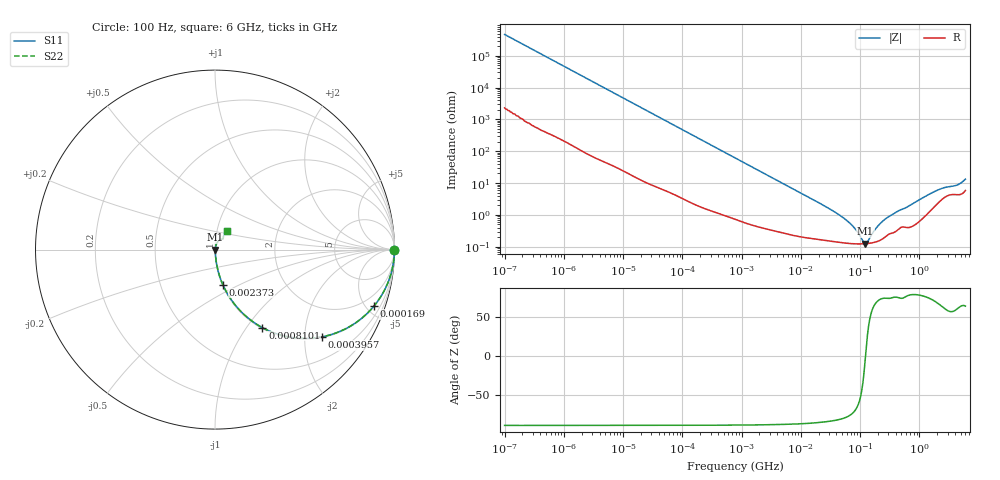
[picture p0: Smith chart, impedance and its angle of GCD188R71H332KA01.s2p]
!Murata Part Number: GCD188R71H332KA01
!These Parameters are Measured in Series Mode Connection
!Data Generated on Jan 08, 2026
!  o--ll--o
!Port1  Port2
!  o------o
!Operation Temp=25[degC], DC Bias Voltage=0[V]
!Freq. Start=100[Hz] Stop=6[GHz] 401[Steps]
# Hz S RI R 50
!Freq.(Hz) S11(Real) S11(Imag) S21(Real) S21(Imag) S12(Real) S12(Imag) S22(Real) S22(Imag)
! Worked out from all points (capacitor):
!   401 points, 100 Hz to 6 GHz, reference 50 ohm
!   read as one part in series: C = 3.4 nF near 109 Hz
!   lowest |Z| = 124 mohm at 122 MHz (marker M1)
!   series resonance near 123.7 MHz, so ESL is about 490 pH
!   S11 on the Smith chart (normalised r, x): 100 Hz: open; 169 kHz: 1.04, -5.66; 395.7 kHz: 1.02, -2.42; 810.1 kHz: 1.01, -1.19; 2.373 MHz: 1.01, -0.41; 6 GHz: 1.12, +0.24
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100  1 -0.000214  1.1e-06 0.000214  1.1e-06 0.000214  1 -0.000214
2008  1 -0.00426  3.67e-05 0.00426  3.67e-05 0.00426  1 -0.00426
40335  0.9924 -0.0842  0.00764 0.0842  0.00764 0.0842  0.9924 -0.0842
169018  0.8871 -0.3129  0.1129 0.3129  0.1129 0.3129  0.8871 -0.3129
395726  0.5941 -0.4864  0.4059 0.4864  0.4059 0.4864  0.5941 -0.4864
774597  0.2811 -0.4437  0.7189 0.4437  0.7189 0.4437  0.2811 -0.4437
810067  0.2637 -0.4347  0.7363 0.4347  0.7363 0.4347  0.2637 -0.4347
1325623  0.1207 -0.3188  0.8793 0.3188  0.8793 0.3188  0.1207 -0.3188
2372521  0.0434 -0.1947  0.9566 0.1947  0.9566 0.1947  0.0434 -0.1947
5311619  0.0109 -0.0906  0.9891 0.0906  0.9891 0.0906  0.0109 -0.0906
1.555665e7  0.00276 -0.0311  0.9972 0.0311  0.9972 0.0311  0.00276 -0.0311
3.64232e7  0.0016 -0.0126  0.9984 0.0126  0.9984 0.0126  0.0016 -0.0126
5.960426e7  0.00133 -0.00654  0.9987 0.00654  0.9987 0.00654  0.00133 -0.00654
8.154455e7  0.00124 -0.00354  0.9988 0.00354  0.9988 0.00354  0.00124 -0.00354
1.115611e8  0.00123 -0.00086  0.9988 0.00086  0.9988 0.00086  0.00123 -0.00086
1.220122e8  0.00124 -0.000115  0.9988 0.000115  0.9988 0.000115  0.00124 -0.000115
1.334425e8  0.00126 0.000632  0.9987 -0.000632  0.9987 -0.000632  0.00126 0.000632
2.088084e8  0.00155 0.00462  0.9984 -0.00462  0.9984 -0.00462  0.00155 0.00462
3.124326e8  0.00258 0.00861  0.9974 -0.00861  0.9974 -0.00861  0.00258 0.00861
1.791126e9  0.02 0.0487  0.98 -0.0487  0.98 -0.0487  0.02 0.0487
4.193612e9  0.046 0.0664  0.954 -0.0664  0.954 -0.0664  0.046 0.0664
6e9  0.067 0.1048  0.933 -0.1048  0.933 -0.1048  0.067 0.1048
